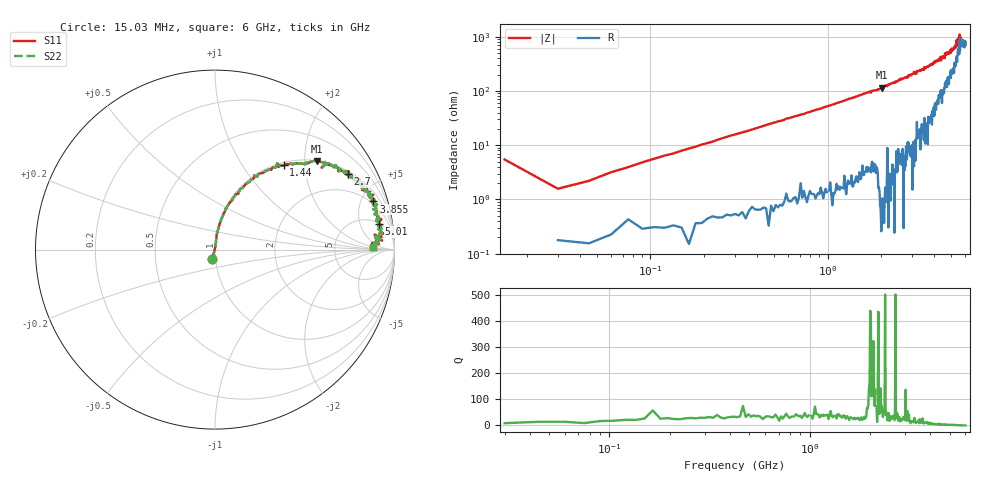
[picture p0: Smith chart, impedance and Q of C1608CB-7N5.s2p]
!	Network	Analyzer	HP8753E.07.74:	Oct	30	2002	Serial	No.	JP38451487
!	Hewlett-Packard
!	27	Aug	2009	16:26:31
!	Frequency	S11	S21	S12	S22
#	HZ	S	RI	R	50
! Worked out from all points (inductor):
!   400 points, 15.03 MHz to 6 GHz, reference 50 ohm
!   read as one part in series: L = 8.31 nH near 45.03 MHz
!   highest Q = 165 at 2.025 GHz (marker M1), where L = 9.02 nH
!   S11 on the Smith chart (normalised r, x): 15.03 MHz: 0.97, -0.10; 1.44 GHz: 1.05, +1.56; 2.7 GHz: 1.11, +3.44; 3.855 GHz: 1.74, +6.27; 5.01 GHz: 5, +10; 6 GHz: 15, +2
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1.502992e7  -0.015 -0.0527  1.02 0.0527  1.02 0.0527  -0.015 -0.0527
3.002985e7  0.00203 0.0156  0.998 -0.0156  0.998 -0.0156  0.00203 0.0156
6.00297e7  0.00349 0.0315  0.997 -0.0315  0.997 -0.0315  0.00349 0.0315
1.200294e8  0.0071 0.0635  0.993 -0.0635  0.993 -0.0635  0.0071 0.0635
2.850286e8  0.0269 0.146  0.973 -0.146  0.973 -0.146  0.0269 0.146
5.850271e8  0.097 0.276  0.903 -0.276  0.903 -0.276  0.097 0.276
1.020025e9  0.228 0.406  0.772 -0.406  0.772 -0.406  0.228 0.406
1.440023e9  0.383 0.471  0.617 -0.471  0.617 -0.471  0.383 0.471
2.01002e9  0.562 0.495  0.438 -0.495  0.438 -0.495  0.562 0.495
2.02502e9  0.568 0.494  0.432 -0.494  0.432 -0.494  0.568 0.494
2.700016e9  0.741 0.422  0.259 -0.422  0.259 -0.422  0.741 0.422
3.015015e9  0.807 0.391  0.193 -0.391  0.193 -0.391  0.807 0.391
3.855011e9  0.883 0.268  0.117 -0.268  0.117 -0.268  0.883 0.268
4.00501e9  0.902 0.251  0.0978 -0.251  0.0978 -0.251  0.902 0.251
5.010005e9  0.914 0.144  0.0856 -0.144  0.0856 -0.144  0.914 0.144
5.385003e9  0.921 0.108  0.0788 -0.108  0.0788 -0.108  0.921 0.108
5.445003e9  0.928 0.0707  0.0722 -0.0707  0.0722 -0.0707  0.928 0.0707
5.535002e9  0.889 0.0836  0.111 -0.0836  0.111 -0.0836  0.889 0.0836
5.565002e9  0.932 0.0508  0.0679 -0.0508  0.0679 -0.0508  0.932 0.0508
5.595002e9  0.893 0.0686  0.107 -0.0686  0.107 -0.0686  0.893 0.0686
5.625002e9  0.912 0.0295  0.0883 -0.0295  0.0883 -0.0295  0.912 0.0295
6e9  0.878 0.0129  0.122 -0.0129  0.122 -0.0129  0.878 0.0129
